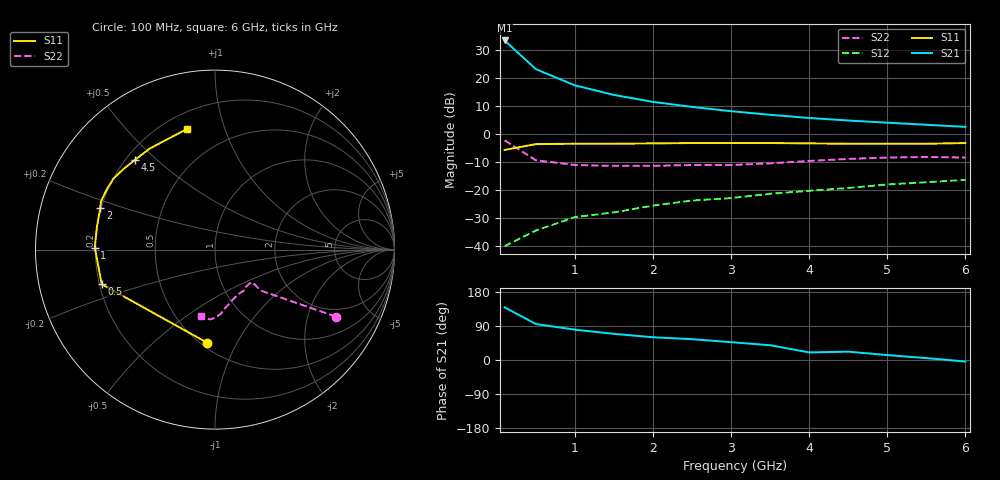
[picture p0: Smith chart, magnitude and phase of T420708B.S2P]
!AT-42070
!S-PARAMETERS at Vce=8V  Ic=35mA.  LAST UPDATED 07-21-92
# ghz s ma r 50
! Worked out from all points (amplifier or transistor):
!   13 points, 100 MHz to 6 GHz, reference 50 ohm
!   highest |S21| = 33.4 dB at 100 MHz (marker M1)
!   |S21| within 3 dB of that: start of sweep to 217.3 MHz
!   unconditionally stable (mu >= 1): 1.046 GHz to 5.874 GHz
!   at 1 GHz: K = 0.98, MSG = 23.5 dB, |S12| = -29.6 dB
!   at 3 GHz: K = 1.23, MAG = 12.6 dB, |S12| = -22.9 dB
!   at 6 GHz: K = 0.99, MSG = 9.5 dB, |S12| = -16.4 dB
!   S11 on the Smith chart (normalised r, x): 100 MHz: 0.54, -0.76; 500 MHz: 0.21, -0.14; 1 GHz: 0.20, +0.01; 2 GHz: 0.20, +0.17; 4.5 GHz: 0.23, +0.42; 6 GHz: 0.29, +0.75
0.1  0.52 -95.0  46.52 139.0  0.01 50.0  0.77 -29.0
0.5  0.66 -163.0  14.33 95.0  0.019 46.0  0.34 -42.0
1  0.67 179.0  7.36 80.0  0.033 51.0  0.28 -41.0
1.5  0.67 169.0  4.97 69.0  0.04 59.0  0.27 -44.0
2  0.68 160.0  3.74 60.0  0.053 59.0  0.27 -51.0
2.5  0.69 157.0  3.04 55.0  0.065 65.0  0.28 -53.0
3  0.69 151.0  2.55 47.0  0.072 65.0  0.28 -62.0
3.5  0.69 145.0  2.2 39.0  0.086 59.0  0.3 -72.0
4  0.68 139.0  1.93 20.0  0.097 60.0  0.33 -80.0
4.5  0.67 132.0  1.74 22.0  0.109 54.0  0.36 -85.0
5  0.67 123.0  1.59 13.0  0.126 50.0  0.38 -90.0
5.5  0.67 113.0  1.46 5.0  0.138 46.0  0.39 -94.0
6  0.69 103.0  1.34 -4.0  0.152 40.0  0.38 -102.0
